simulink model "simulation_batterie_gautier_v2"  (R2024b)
settings: Solver=VariableStepAuto  StartTime=0.0  StopTime=280000  FixedStep=1  RelTol=1e-3
model workspace (MAT data in the model file):
  DOD = 0.5
undefined symbols (not defined in the file): Hydride, Ion, Lithium, Metal, Nickel
libraries: spsBatteryLib x3, spsParallelRLCLoadLib x3, sps_lib x1

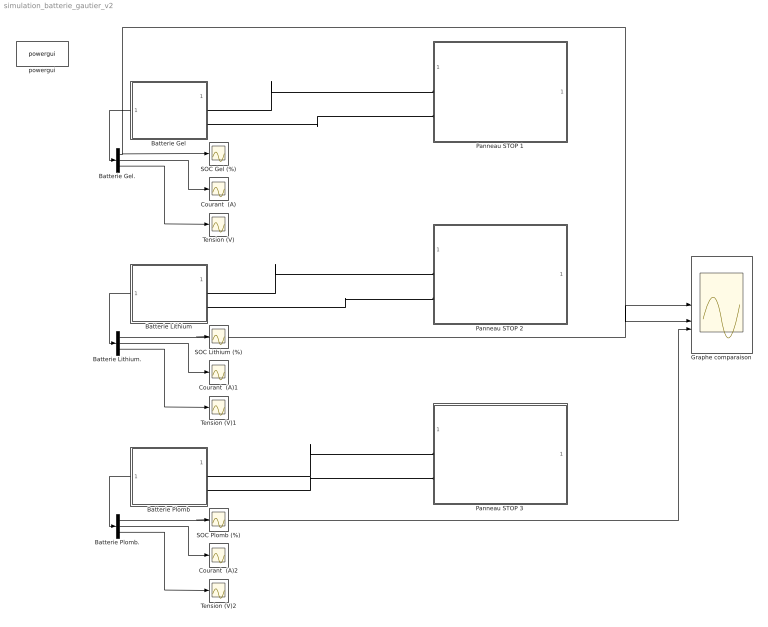
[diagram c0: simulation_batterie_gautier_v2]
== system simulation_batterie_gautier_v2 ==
  Batterie Gel : Subsystem
  Batterie Gel. : Demux  Outputs=3
  Batterie Lithium : Subsystem
  Batterie Lithium. : Demux  Outputs=3
  Batterie Plomb : Subsystem
  Batterie Plomb. : Demux  Outputs=3
  Courant  (A) : Scope
  Courant  (A)1 : Scope
  Courant  (A)2 : Scope
  Graphe comparaison : Scope  NumInputPorts=3
  Panneau STOP 1 : Subsystem
  Panneau STOP 2 : Subsystem
  Panneau STOP 3 : Subsystem
  SOC Gel (%) : Scope
  SOC Lithium (%) : Scope
  SOC Plomb (%) : Scope
  Tension (V) : Scope
  Tension (V)1 : Scope
  Tension (V)2 : Scope
  powergui : sps_lib/powergui  Priority=1  SimulationMode=Continuous  SampleTime=50e-6  frequency=60  Iterations=50  frequencyindice=0  Pbase=100e6  ErrMax=1e-4  UnitsV=kV  UnitsW=MW  buscounter=0  FunctionMessages=off  echomessages=off  EnableUseOfTLC=off  CurrentSourceSwitches=off  DisableSnubberDevices=off  DisableRonSwitches=off  DisableVfSwitches=off  DisplayEquations=off  AutomaticDiscreteSolvers=off  SolverType=Tustin/Backward Euler (TBE)  Interpol=off  ExternalGateDelay=off  methode=off  Ts=100  x0status=blocks  SPID=on  SwTol=0  HookPort=off  NonlinearTolerance=1e-4  nMaxIteration=100  ContinueOnMaxIteration=off  RestoreLinks=warning  ResistiveCurrentMeasurement=off  Frange=[0:2:500]  Ylog=off  Xlog=on  ShowGrid=off  save=off  variable=ZData  structure=0  ZoomFFT=off  StartTime=0.0  cycles=1  DisplayStyle=1  fundamental=60  FreqAxis=off  MaxFrequency=1000  frequencyindicesteady=1  RmsSteady=1  display=off
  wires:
  Batterie Gel./1 -> SOC Gel (%)/1, Graphe comparaison/1
  Batterie Gel./2 -> Courant  (A)/1
  Batterie Gel./3 -> Tension (V)/1
  Batterie Gel/1(m) -> Batterie Gel./1
  Batterie Lithium./2 -> Courant  (A)1/1
  Batterie Lithium./1 -> SOC Lithium (%)/1, Graphe comparaison/2
  Batterie Lithium./3 -> Tension (V)1/1
  Batterie Lithium/1(m) -> Batterie Lithium./1
  Batterie Plomb./2 -> Courant  (A)2/1
  Batterie Plomb./1 -> SOC Plomb (%)/1, Graphe comparaison/3
  Batterie Plomb./3 -> Tension (V)2/1
  Batterie Plomb/1(m) -> Batterie Plomb./1
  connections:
  Batterie Gel/LConn1 -- Panneau STOP 1/LConn1
  Panneau STOP 1/LConn2 -- Batterie Gel/LConn2
  Batterie Lithium/LConn1 -- Panneau STOP 2/LConn1
  Batterie Lithium/LConn2 -- Panneau STOP 2/LConn2
  Batterie Plomb/LConn1 -- Panneau STOP 3/LConn1
  Batterie Plomb/LConn2 -- Panneau STOP 3/LConn2

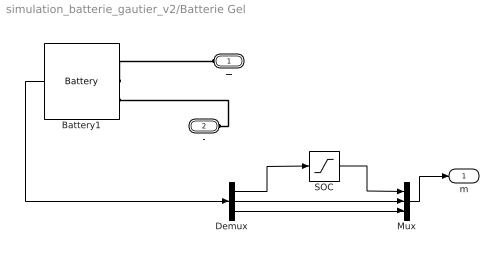
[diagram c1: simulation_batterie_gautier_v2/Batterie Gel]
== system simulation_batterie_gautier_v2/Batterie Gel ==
  Battery1 : spsBatteryLib/Battery  BatType=Nickel-Metal-Hydride  NomV=12  NomQ=60  SOC=100  Batt_Tr=30  PresetModel=on  MaxQ=64.6154  MinV=9  FullV=14.1356  Dis_rate=12  R=0.002  Normal_OP=57.6923  expZone="[13.0169           12]"
  Demux : Demux  Outputs=3
  Mux : Mux  Inputs=3
  SOC : Saturate  UpperLimit=inf  LowerLimit=40
  + : PMIOPort  Side=Left
  - : PMIOPort  Port=2  Side=Left
  m : Outport
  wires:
  Battery1/1 -> Demux/1
  Demux/1 -> SOC/1
  SOC/1 -> Mux/1
  Mux/1 -> m/1
  Demux/2 -> Mux/2
  Demux/3 -> Mux/3
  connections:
  Battery1/LConn1 -- +/RConn1
  -/RConn1 -- Battery1/LConn2

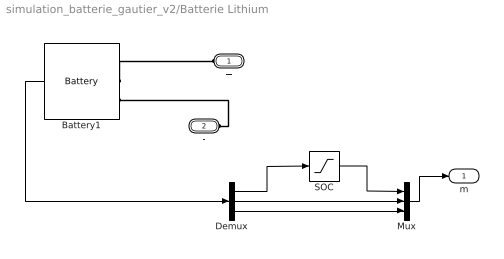
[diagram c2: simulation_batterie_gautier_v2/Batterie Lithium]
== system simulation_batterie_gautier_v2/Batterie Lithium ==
  Battery1 : spsBatteryLib/Battery  BatType=Lithium-Ion  NomV=12.8  NomQ=57  SOC=100  Batt_Tr=30  PresetModel=on  MaxQ=57  MinV=9.6  FullV=14.899  Dis_rate=24.7826  R=0.0022456  Normal_OP=51.5478  expZone="[13.8289      2.80043]"
  Demux : Demux  Outputs=3
  Mux : Mux  Inputs=3
  SOC : Saturate  UpperLimit=inf  LowerLimit=20
  + : PMIOPort  Side=Left
  - : PMIOPort  Port=2  Side=Left
  m : Outport
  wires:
  Battery1/1 -> Demux/1
  Demux/1 -> SOC/1
  SOC/1 -> Mux/1
  Mux/1 -> m/1
  Demux/2 -> Mux/2
  Demux/3 -> Mux/3
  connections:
  Battery1/LConn1 -- +/RConn1
  -/RConn1 -- Battery1/LConn2

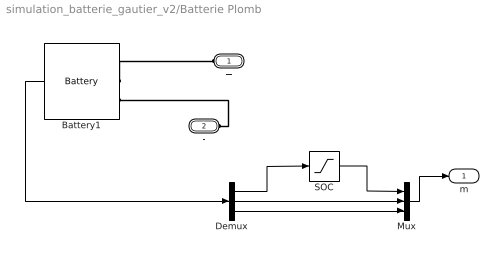
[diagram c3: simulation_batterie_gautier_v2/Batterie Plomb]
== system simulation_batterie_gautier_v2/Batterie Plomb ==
  Battery1 : spsBatteryLib/Battery  BatType=Lithium-Ion  NomV=12  NomQ=62  SOC=100  Batt_Tr=30  PresetModel=on  MaxQ=62  MinV=9  FullV=13.9678  Dis_rate=26.9565  R=0.0019355  Normal_OP=56.0696  expZone="[12.9646      3.04609]"
  Demux : Demux  Outputs=3
  Mux : Mux  Inputs=3
  SOC : Saturate  UpperLimit=inf  LowerLimit=50
  + : PMIOPort  Side=Left
  - : PMIOPort  Port=2  Side=Left
  m : Outport
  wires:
  Battery1/1 -> Demux/1
  Demux/1 -> SOC/1
  SOC/1 -> Mux/1
  Mux/1 -> m/1
  Demux/2 -> Mux/2
  Demux/3 -> Mux/3
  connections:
  Battery1/LConn1 -- +/RConn1
  -/RConn1 -- Battery1/LConn2

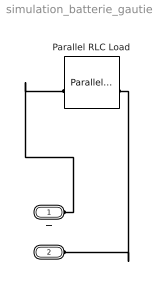
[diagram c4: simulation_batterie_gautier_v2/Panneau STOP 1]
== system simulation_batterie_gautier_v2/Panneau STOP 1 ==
  Parallel RLC Load : spsParallelRLCLoadLib/Parallel RLC Load  LConnTagsString=a  RConnTagsString=__new0  NominalVoltage=12  NominalFrequency=0.001  ActivePower=(16*8+8*4)/24  InductivePower=0  CapacitivePower=0  Setx0=off  InitialVoltage=0  SetiL0=off  InitialCurrent=0  Measurements=None  LoadType=constant PQ
  + : PMIOPort  Side=Left
  - : PMIOPort  Port=2  Side=Left
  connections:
  +/RConn1 -- Parallel RLC Load/LConn1
  Parallel RLC Load/RConn1 -- -/RConn1

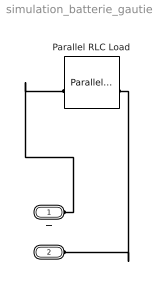
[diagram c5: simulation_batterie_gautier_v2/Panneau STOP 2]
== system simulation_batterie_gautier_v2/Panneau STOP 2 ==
  Parallel RLC Load : spsParallelRLCLoadLib/Parallel RLC Load  LConnTagsString=a  RConnTagsString=__new0  NominalVoltage=12  NominalFrequency=0.001  ActivePower=(16*8+8*4)/24  InductivePower=0  CapacitivePower=0  Setx0=off  InitialVoltage=0  SetiL0=off  InitialCurrent=0  Measurements=None  LoadType=constant PQ
  + : PMIOPort  Side=Left
  - : PMIOPort  Port=2  Side=Left
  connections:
  +/RConn1 -- Parallel RLC Load/LConn1
  Parallel RLC Load/RConn1 -- -/RConn1

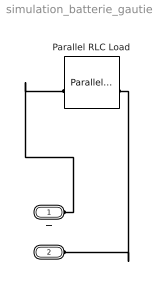
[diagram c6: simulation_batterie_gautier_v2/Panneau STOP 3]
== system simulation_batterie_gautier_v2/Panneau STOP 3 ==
  Parallel RLC Load : spsParallelRLCLoadLib/Parallel RLC Load  LConnTagsString=a  RConnTagsString=__new0  NominalVoltage=12  NominalFrequency=0.001  ActivePower=(16*8+8*4)/24  InductivePower=0  CapacitivePower=0  Setx0=off  InitialVoltage=0  SetiL0=off  InitialCurrent=0  Measurements=None  LoadType=constant PQ
  + : PMIOPort  Side=Left
  - : PMIOPort  Port=2  Side=Left
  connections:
  +/RConn1 -- Parallel RLC Load/LConn1
  Parallel RLC Load/RConn1 -- -/RConn1
